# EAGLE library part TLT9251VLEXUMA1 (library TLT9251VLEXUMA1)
CAN Interface IC Source: Datasheet
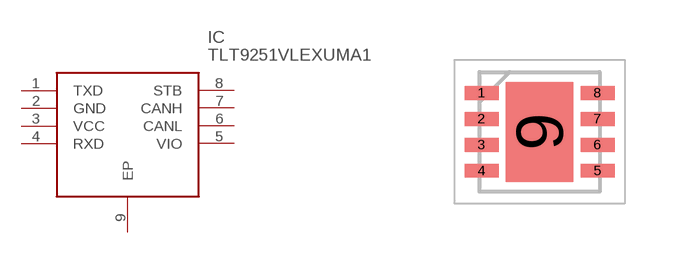
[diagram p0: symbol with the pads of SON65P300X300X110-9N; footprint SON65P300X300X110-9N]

Designator prefix IC

## TLT9251VLEXUMA1 (Arrow_Part_Number: TLT9251VLEXUMA1; Arrow_Price-Stock: https://www.arrow.com/en/products/tlt9251vlexuma1/infineon-technologies-ag?region=nac; Description: CAN Interface IC; Height: 1.1mm; Manufacturer_Name: Infineon; Manufacturer_Part_Number: TLT9251VLEXUMA1; Mouser_Part_Number: 726-TLT9251VLEXUMA1; Mouser_Price-Stock: https://www.mouser.co.uk/ProductDetail/Infineon-Technologies/TLT9251VLEXUMA1?qs=W%2FMpXkg%252BdQ5zGtp9sfvtfA%3D%3D)  [SON65P300X300X110-9N]
1  TXD
2  GND
3  VCC
4  RXD
5  VIO
6  CANL
7  CANH
8  STB
9  EP

## Footprint SON65P300X300X110-9N (pad centres in mm)
PG-TSON-8-
smd 0.85 x 0.35: 1 -1.45,0.975; 2 -1.45,0.325; 3 -1.45,-0.325; 4 -1.45,-0.975; 5 1.45,-0.975; 6 1.45,-0.325; 7 1.45,0.325; 8 1.45,0.975
smd 1.68 x 2.5: 9 0,0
